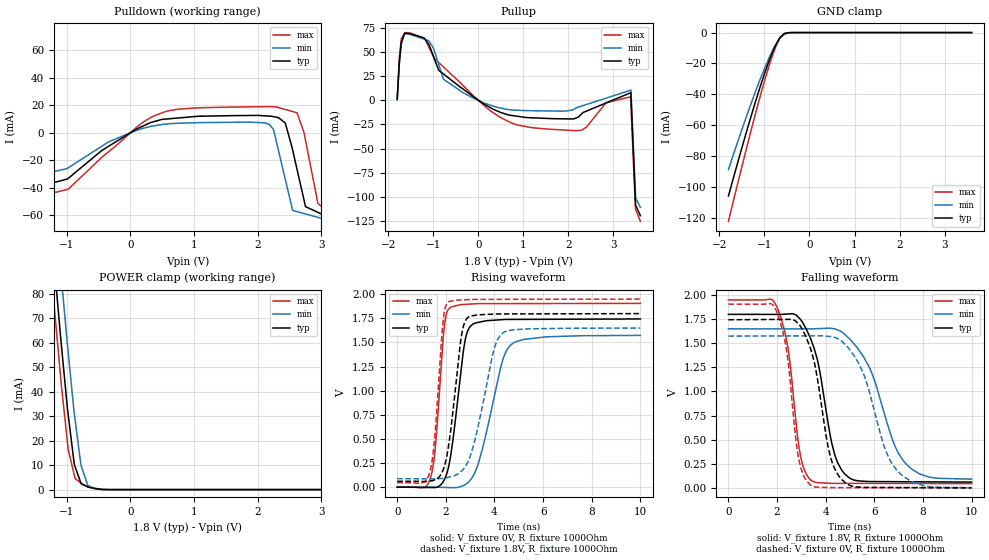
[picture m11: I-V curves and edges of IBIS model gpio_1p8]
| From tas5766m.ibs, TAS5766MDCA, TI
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|   gpio_1p8 Model
[Model]   gpio_1p8
Model_type   I/O
Polarity   Non-Inverting
Enable   Active-Low
Vinl = 0.54
Vinh = 1.26
Vmeas = 0.9
Vref = 0
Cref = 1pF
Rref = 1000000
|   typ   min   max
C_comp   1.487pF   1.458pF   1.501pF
[Voltage Range]   1.8   1.65   1.95
[Temperature Range]   27   105   -25
[Pullup Reference]   1.8   1.65   1.95
[Pulldown Reference]   -0   -0   -0
[Power Clamp Reference]   1.8   1.65   1.95
[GND Clamp Reference]   -0   -0   -0
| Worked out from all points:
|   slope of the pulldown table from 0 to 0.27 V, typ, clamps not added: 41.9 ohm
|   slope of the pullup table from 0 to 0.27 V, typ, clamps not added: 34.4 ohm
|   GND clamp passes 1 mA (typ) near -0.57 V on its own axis
|   POWER clamp passes 1 mA (typ) near -0.66 V on its own axis
|   falling waveform, V_fixture 1.8V, R_fixture 1000Ohm: 20-80 % time 787ps typ, 1.3ns min, 537ps max; typ from 1.8 V to 0.06 V
|   rising waveform, V_fixture 0V, R_fixture 1000Ohm: 20-80 % time 501ps typ, 860ps min, 331ps max; typ from 0 V to 1.74 V
|   rising waveform, V_fixture 1.8V, R_fixture 1000Ohm: 20-80 % time 480ps typ, 794ps min, 326ps max; typ from 0.06 V to 1.8 V
|   falling waveform, V_fixture 0V, R_fixture 1000Ohm: 20-80 % time 736ps typ, 1.17ns min, 514ps max; typ from 1.74 V to 0 V
[Pulldown]
|   Voltage   I(typ)   I(min)   I(max)
-1.8V     -18.87mA   -14.29mA   -22.86mA
-1.709V   -38.03mA   -24.52mA   -45.94mA
-1.514V   -40.09mA   -31.67mA   -47.45mA
549.5mV   9.988mA    6.335mA    15.44mA
2.107V    12.39mA    7.278mA    19.06mA
2.293V    11.39mA    -6.132mA   18.88mA
2.55V     -12.55mA   -56.54mA   15.49mA
2.752V    -53.77mA   -59.13mA   -5.426mA
2.947V    -57.98mA   -61.63mA   -51.48mA
3.382V    -67.39mA   -67.22mA   -68.3mA
3.491V    241mA      311.3mA    184mA
3.6V      283.7mA    359.8mA    218.7mA
[GND Clamp]
|   Voltage   I(typ)   I(min)   I(max)
-1.8V     -105.9mA   -88.79mA   -122.2mA
-1.526V   -77.2mA    -64.95mA   -89.74mA
-1.31V    -55.47mA   -46.98mA   -64.86mA
-1.094V   -35.02mA   -30.15mA   -41.18mA
-973.6mV  -24.51mA   -21.51mA   -28.77mA
-865.6mV  -15.91mA   -14.42mA   -18.57mA
-757.6mV  -8.516mA   -8.254mA   -9.666mA
-649.6mV  -3.097mA   -3.535mA   -3.115mA
-541.6mV  -521.7uA   -891.9uA   -362.1uA
-343.1mV  -3.165uA   -10.49uA   -2.518uA
3.6V      0A         0A         0A
[Pullup]
|   Voltage   I(typ)   I(min)   I(max)
-1.8V     1.162mA    800.1uA    1.539mA
-1.709V   60.48mA    58.45mA    64.49mA
-1.622V   70.03mA    69.37mA    70.69mA
-1.099V   58.46mA    62.21mA    55.63mA
-775.1mV  27.66mA    22.23mA    34.91mA
-343.1mV  12.09mA    8.282mA    15.79mA
847.2mV   -16.28mA   -10.09mA   -25.23mA
2.293V    -14.1mA    -5.848mA   -31.08mA
2.838V    -2.602mA   2.419mA    -2.365mA
3.382V    7.998mA    10.69mA    3.848mA
3.491V    -105.5mA   -97.34mA   -113mA
3.6V      -119.9mA   -111.3mA   -125.8mA
[POWER Clamp]
|   Voltage   I(typ)   I(min)   I(max)
-1.8V     283.3mA    311.2mA    266.4mA
-1.207V   96.06mA    124.1mA    79.07mA
-1.19V    90.85mA    118.8mA    73.77mA
-1.099V   64.09mA    91.62mA    47.73mA
-1.082V   59.21mA    86.58mA    42.71mA
-973.6mV  30.48mA    55.88mA    16.29mA
-878.5mV  10.27mA    31.08mA    5.906mA
-865.6mV  9.338mA    28.48mA    4.507mA
-770.5mV  2.394mA    9.783mA    2.613mA
-667.1mV  1.068mA    1.694mA    1.223mA
-559.1mV  542.6uA    410.6uA    348.9uA
3.6V      0A         0A         0A
[Ramp]
R_load = 1000
|   typ   min   max
dV/dt_r   1.0465/5.00691e-10   0.944178/8.58113e-10   1.14355/3.30974e-10
dV/dt_f   1.04404/7.82813e-10   0.935761/1.29852e-09   1.14349/5.36547e-10
[Falling Waveform]
V_fixture = 1.8V
V_fixture_min = 1.65V
V_fixture_max = 1.95V
R_fixture = 1000Ohm
C_fixture = 0F
|   Time   V(typ)   V(min)   V(max)
0s        1.8V       1.65V      1.95V
1.98ns    1.8V       1.65V      1.884V
2.458ns   1.804V     1.65V      1.439V
2.972ns   1.744V     1.65V      320.7mV
3.378ns   1.548V     1.65V      82.43mV
4.26ns    452.7mV    1.654V     46.96mV
4.768ns   147.7mV    1.596V     46.71mV
5.799ns   65.75mV    1.248V     46.21mV
7.285ns   63.69mV    253.6mV    45.49mV
10ns      59.94mV    90.4mV     44.17mV
[Rising Waveform]
V_fixture = 0V
V_fixture_min = 0V
V_fixture_max = 0V
R_fixture = 1000Ohm
C_fixture = 0F
|   Time   V(typ)   V(min)   V(max)
0s        1.664nV    40.86nV    825.3pV
1.364ns   -4.646mV   631.9uV    91.77mV
1.557ns   -5.305mV   -779.9uV   388mV
1.942ns   79.48mV    -3.812mV   1.676V
2.165ns   277.4mV    -5.57mV    1.86V
2.783ns   1.509V     23.69mV    1.895V
3.111ns   1.69V      112mV      1.9V
4.297ns   1.737V     1.281V     1.903V
4.664ns   1.739V     1.473V     1.904V
10ns      1.744V     1.574V     1.906V
[Rising Waveform]
V_fixture = 1.8V
V_fixture_min = 1.65V
V_fixture_max = 1.95V
R_fixture = 1000Ohm
C_fixture = 0F
|   Time   V(typ)   V(min)   V(max)
0s        59.83mV    87.22mV    44.11mV
1.333ns   62.75mV    85.52mV    150.1mV
1.521ns   72.81mV    85.28mV    460.2mV
1.89ns    179.4mV    91.08mV    1.73V
2.089ns   391mV      101.6mV    1.917V
2.625ns   1.54V      162.9mV    1.941V
2.911ns   1.761V     264.8mV    1.944V
3.949ns   1.794V     1.398V     1.948V
4.355ns   1.796V     1.601V     1.948V
10ns      1.8V       1.65V      1.95V
[Falling Waveform]
|Gnd
V_fixture = 0V
V_fixture_min = 0V
V_fixture_max = 0V
R_fixture = 1000Ohm
C_fixture = 0F
|   Time   V(typ)   V(min)   V(max)
0s        1.744V     1.574V     1.906V
1.942ns   1.747V     1.576V     1.851V
2.399ns   1.748V     1.576V     1.411V
2.901ns   1.697V     1.577V     285.4mV
3.378ns   1.442V     1.577V     27.82mV
4.108ns   414.5mV    1.572V     3.175mV
4.668ns   84.06mV    1.52V      1.949mV
5.518ns   5.283mV    1.206V     1.648mV
6.913ns   3.592mV    186.8mV    1.153mV
10ns      96.19uV    1.633mV    57.44uV
